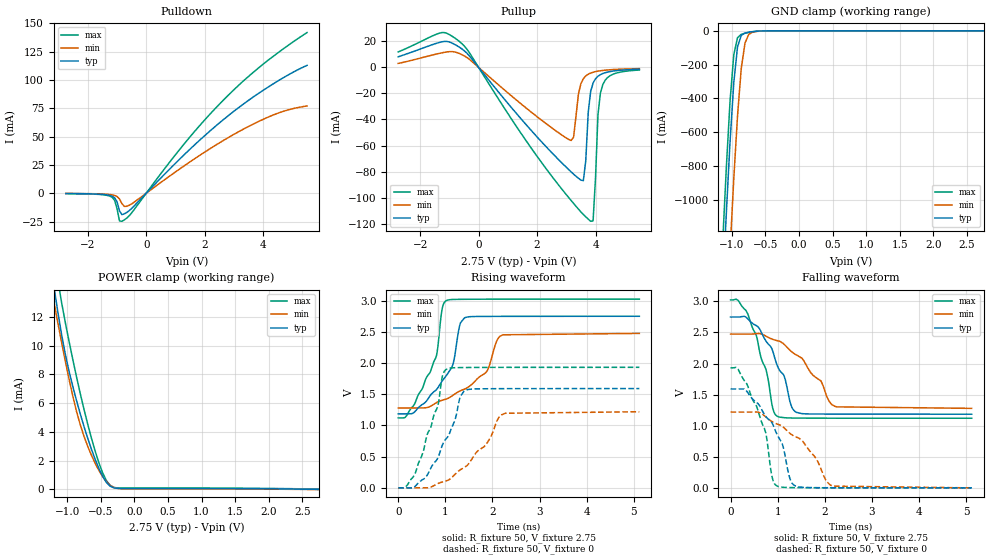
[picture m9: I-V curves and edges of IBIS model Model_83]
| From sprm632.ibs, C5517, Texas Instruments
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| Model based on original model for BC3340CTSCHYPD
|   Sub model SR0_VDD_SR1_VDD_PD_ON_COM_2P75
[model]   Model_83
|[Description]  [2.75V-I/O-PD-X, COM]
|   PD,COM,
|[Input Load]   PD
|[Output Drive]
|Voltage   2.75V
|Mode   I/O
Model_type   I/O
Polarity   Non-Inverting
Enable   Active-Low
Vinl =  0.7
Vinh =  1.7
Cref =  15.0000pF
Rref =  100.0000M
Vref =  0V
Vmeas =  1.375
C_comp   2.1456989p   2.0494201p   2.2784851p
[Model Spec]
Vinl   0.7   0.7   0.7
Vinh   1.7   1.7   1.7
[Temperature Range]   25   105   -10
[Voltage Range]   2.75   2.475   3.025
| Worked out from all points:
|   slope of the pulldown table from 0 to 0.412 V, typ, clamps not added: 37.1 ohm
|   slope of the pullup table from 0 to 0.412 V, typ, clamps not added: 35.9 ohm
|   GND clamp passes 1 mA (typ) near -0.57 V on its own axis
|   POWER clamp passes 1 mA (typ) near -0.48 V on its own axis
|   rising waveform, R_fixture 50, V_fixture 2.75: 20-80 % time 563ps typ, 807ps min, 459ps max; typ from 1.19 V to 2.75 V
|   rising waveform, R_fixture 50, V_fixture 0: 20-80 % time 567ps typ, 804ps min, 464ps max; typ from 0 V to 1.59 V
|   falling waveform, R_fixture 50, V_fixture 2.75: 20-80 % time 532ps typ, 786ps min, 413ps max; typ from 2.75 V to 1.19 V
|   falling waveform, R_fixture 50, V_fixture 0: 20-80 % time 554ps typ, 830ps min, 430ps max; typ from 1.59 V to 0 V
[POWER_clamp]
-2.75V    68.54mA    53.4mA     84.13mA
-1.25V    15.8mA     14.35mA    18.37mA
-1.194V   14.01mA    12.94mA    16.33mA
-1.139V   12.31mA    11.56mA    14.54mA
-1.083V   10.75mA    10.21mA    12.98mA
-972.2mV  8.203mA    7.648mA    10.28mA
-805.6mV  5.244mA    4.485mA    6.656mA
-694.4mV  3.547mA    2.986mA    4.521mA
-527.8mV  1.441mA    1.31mA     1.833mA
-361.1mV  223.7uA    277.8uA    276.3uA
-138.9mV  61.83uA    37.73uA    92.51uA
2.75V     -8.84nA    -15.87uA   21.46uA
[Pulldown]
-2.75V    -308.5uA   -227.6uA   -371.5uA
-1.25V    -1.93mA    -1.163mA   -2.58mA
-1.083V   -4.054mA   -1.991mA   -6.245mA
-1V       -7.547mA   -2.954mA   -13.7mA
-916.7mV  -15.6mA    -5.046mA   -24.44mA
-833.3mV  -18.95mA   -9.139mA   -24.82mA
-750mV    -18.23mA   -11.68mA   -23.55mA
-500mV    -13.48mA   -9.45mA    -17.38mA
1.333V    34.87mA    24.79mA    44.69mA
2.583V    63.77mA    45.72mA    80.76mA
4.25V     95.04mA    68.08mA    119mA
5.5V      112.9mA    77.06mA    141.9mA
[Pullup]
-2.75V    8.15mA     3.088mA    11.86mA
-1.25V    19.65mA    11.21mA    26.74mA
-583.3mV  14.38mA    9.918mA    18.47mA
3.167V    -80.24mA   -56.1mA    -102.2mA
3.583V    -86.93mA   -8.662mA   -112.9mA
3.667V    -71.56mA   -6.559mA   -114.7mA
3.833V    -18.5mA    -4.358mA   -118.1mA
3.917V    -11.98mA   -3.72mA    -117.8mA
4V        -8.725mA   -3.242mA   -84.8mA
4.083V    -6.819mA   -2.87mA    -36.49mA
4.25V     -4.711mA   -2.331mA   -13.16mA
5.5V      -1.388mA   -959.6uA   -2.008mA
[GND_clamp]
-2.75V    -17.03A    -17.67A    -16.78A
-1.139V   -1.54A     -2.231A    -1.261A
-1.083V   -1.078A    -1.755A    -809.5mA
-1.028V   -655mA     -1.299A    -415mA
-972.2mV  -306mA     -874.1mA   -141.2mA
-916.7mV  -94.94mA   -503mA     -40.42mA
-861.1mV  -27.25mA   -223.2mA   -20.89mA
-805.6mV  -13.1mA    -72.24mA   -14.24mA
-750mV    -8.089mA   -21.21mA   -9.46mA
-694.4mV  -4.87mA    -8.039mA   -5.651mA
-638.9mV  -2.576mA   -3.815mA   -2.865mA
2.75V     61.47uA    87.87uA    92.23uA
[Ramp]
dV/dt_f 0.94544855/0.53821736n 0.72302941/0.79618079n  1.1499934/0.41706488n
dV/dt_r 0.95570412/0.56851356n  0.7324342/0.80577395n  1.1597681/0.46430937n
R_load = 50
[Rising Waveform]
R_fixture = 50
V_fixture = 2.75
V_fixture_min = 2.475
V_fixture_max = 3.025
0s        1.186V     1.28V      1.121V
675.6ps   1.473V     1.303V     1.849V
813.4ps   1.576V     1.365V     2.123V
933.3ps   1.711V     1.404V     2.87V
1.01ns    1.787V     1.421V     2.995V
1.157ns   1.964V     1.481V     3.018V
1.411ns   2.725V     1.583V     3.021V
1.865ns   2.746V     1.849V     3.022V
2.223ns   2.747V     2.452V     3.023V
5.12ns    2.749V     2.474V     3.023V
[Rising Waveform]
R_fixture = 50
V_fixture = 0
V_fixture_min = 0
V_fixture_max = 0
0s        0V         0V         0V
363.8ps   28.86mV    0V         238.6mV
838.2ps   475mV      66.62mV    1.304V
929.1ps   668.1mV    92.67mV    1.758V
1.014ns   784.1mV    109.9mV    1.895V
1.399ns   1.552V     324.1mV    1.927V
1.851ns   1.587V     680.9mV    1.93V
2.127ns   1.589V     1.117V     1.93V
2.275ns   1.589V     1.195V     1.93V
5.12ns    1.591V     1.219V     1.931V
[Falling Waveform]
R_fixture = 50
V_fixture = 2.75
V_fixture_min = 2.475
V_fixture_max = 3.025
0s        2.749V     2.474V     3.024V
367.6ps   2.719V     2.474V     2.797V
605.5ps   2.571V     2.484V     2.238V
777.1ps   2.336V     2.431V     1.825V
897.4ps   2.197V     2.389V     1.277V
987.5ps   1.976V     2.37V      1.153V
1.365ns   1.23V      2.152V     1.123V
1.919ns   1.188V     1.72V      1.121V
2.204ns   1.186V     1.315V     1.121V
5.12ns    1.185V     1.28V      1.12V
[Falling Waveform]
R_fixture = 50
V_fixture = 0
V_fixture_min = 0
V_fixture_max = 0
0s        1.591V     1.219V     1.932V
162.3ps   1.591V     1.219V     1.906V
549.2ps   1.376V     1.221V     1.319V
749.6ps   1.146V     1.141V     880.2mV
901ps     1.015V     1.057V     121mV
1.008ns   829.1mV    1.022V     23.24mV
1.272ns   125.9mV    870.4mV    4.612mV
1.415ns   20.1mV     810.9mV    3.312mV
2.168ns   1.795mV    27.8mV     922.5uV
5.12ns    17.08uV    164.1uV    0V
